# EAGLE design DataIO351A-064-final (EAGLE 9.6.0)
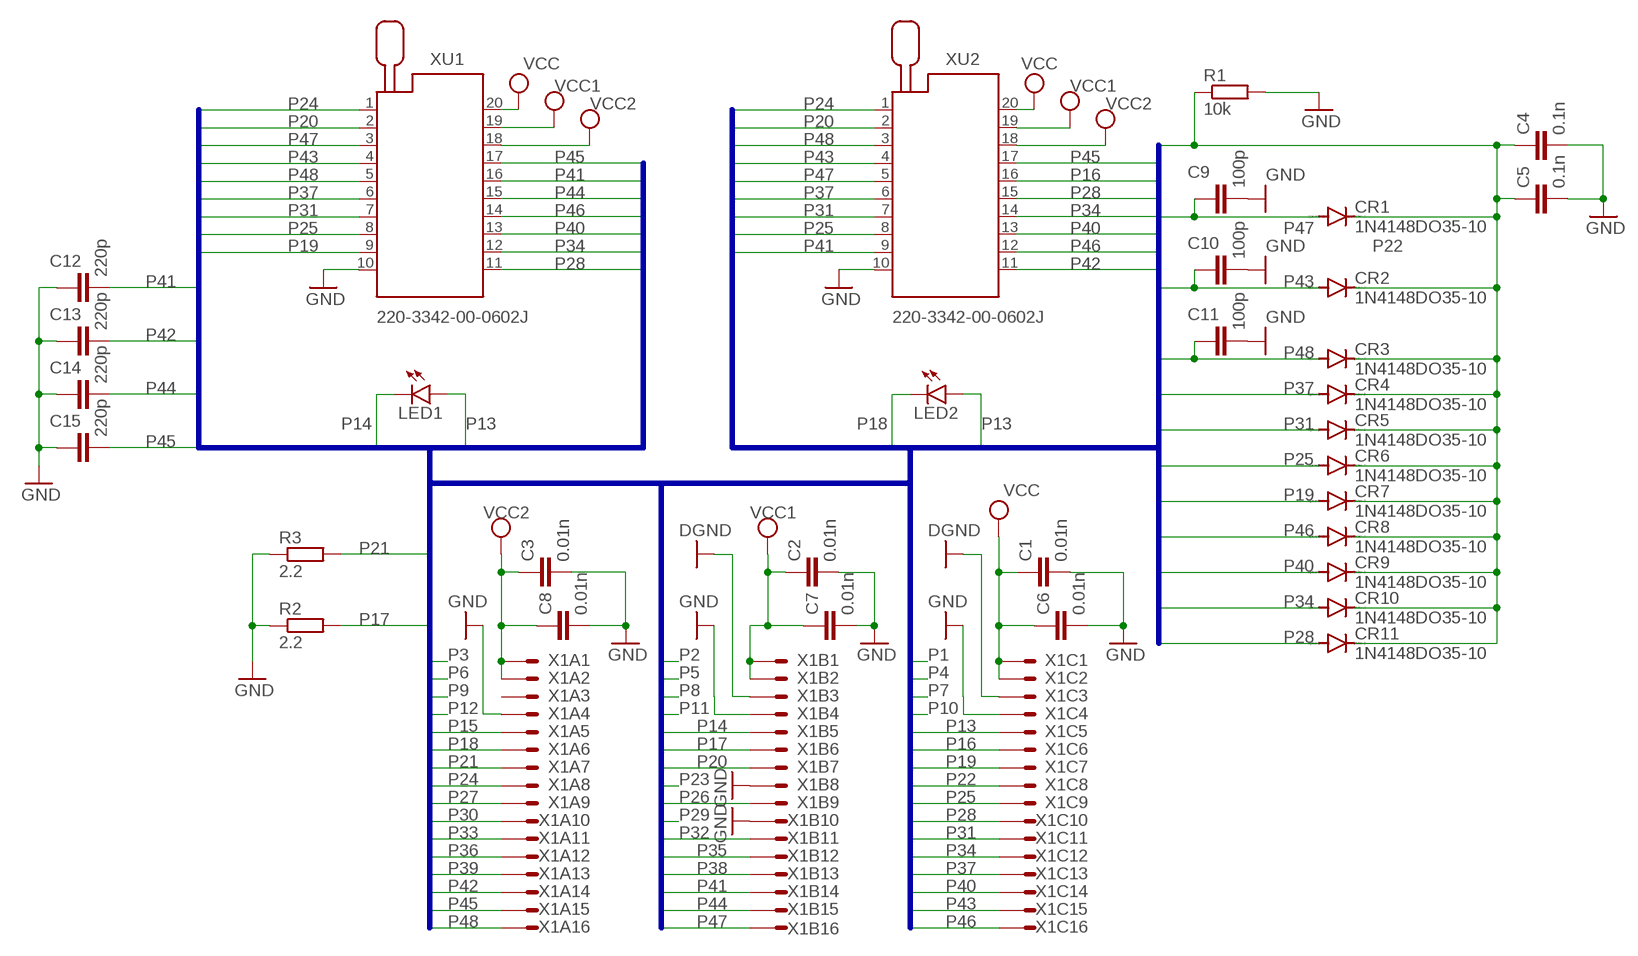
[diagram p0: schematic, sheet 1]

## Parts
C1  0.01n  C-EU050-025X075  [C050-025X075]
C2  0.01n  C-EU050-025X075  [C050-025X075]
C3  0.01n  C-EU050-025X075  [C050-025X075]
C4  0.1n  C-EU050-025X075  [C050-025X075]
C5  0.1n  C-EU050-025X075  [C050-025X075]
C6  0.01n  C-EU050-025X075  [C050-025X075]
C7  0.01n  C-EU050-025X075  [C050-025X075]
C8  0.01n  C-EU050-025X075  [C050-025X075]
C9  100p  C-EU050-025X075  [C050-025X075]
C10  100p  C-EU050-025X075  [C050-025X075]
C11  100p  C-EU050-025X075  [C050-025X075]
C12  220p  C-EU050-025X075  [C050-025X075]
C13  220p  C-EU050-025X075  [C050-025X075]
C14  220p  C-EU050-025X075  [C050-025X075]
C15  220p  C-EU050-025X075  [C050-025X075]
CR1  1N4148DO35-10  [DO35-10]
CR2  1N4148DO35-10  [DO35-10]
CR3  1N4148DO35-10  [DO35-10]
CR4  1N4148DO35-10  [DO35-10]
CR5  1N4148DO35-10  [DO35-10]
CR6  1N4148DO35-10  [DO35-10]
CR7  1N4148DO35-10  [DO35-10]
CR8  1N4148DO35-10  [DO35-10]
CR9  1N4148DO35-10  [DO35-10]
CR10  1N4148DO35-10  [DO35-10]
CR11  1N4148DO35-10  [DO35-10]
LED1  LED5MM  [LED5MM]
LED2  LED5MM  [LED5MM]
R1  10k  R-EU_V234/12  [V234/12]
R2  2.2  R-EU_V234/12  [V234/12]
R3  2.2  R-EU_V234/12  [V234/12]
X1  MAC48SHE  [MAC48SH]
XU1  220-3342-00-0602J  [220-3342-00-0602J]
XU2  220-3342-00-0602J  [220-3342-00-0602J]

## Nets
DGND: X1.B3 X1.C3
GND: C1.2 C2.2 C3.2 C4.2 C5.2 C6.2 C7.2 C8.2 C9.2 C10.2 C11.2 C12.1 C13.1 C14.1 C15.1 R1.2 R2.1 R3.1 X1.A4 X1.B4 X1.B8 X1.B10 X1.C4 XU1.10 XU2.10
P13: LED1.A LED2.A X1.C5
P14: LED1.K(C) X1.B5
P15: X1.A5
P16: X1.C6 XU2.16
P17: R2.2 X1.B6
P18: LED2.K(C) X1.A6
P19: CR7.A X1.C7 XU1.9
P20: X1.B7 XU1.2 XU2.2
P21: R3.2 X1.A7
P22: C4.1 C5.1 CR1.C CR2.C CR3.C CR4.C CR5.C CR6.C CR7.C CR8.C CR9.C CR10.C CR11.C R1.1 X1.C8
P24: X1.A8 XU1.1 XU2.1
P25: CR6.A X1.C9 XU1.8 XU2.8
P26: X1.B9
P27: X1.A9
P28: CR11.A X1.C10 XU1.11 XU2.15
P30: X1.A10
P31: CR5.A X1.C11 XU1.7 XU2.7
P32: X1.B11
P33: X1.A11
P34: CR10.A X1.C12 XU1.12 XU2.14
P35: X1.B12
P36: X1.A12
P37: CR4.A X1.C13 XU1.6 XU2.6
P38: X1.B13
P39: X1.A13
P40: CR9.A X1.C14 XU1.13 XU2.13
P41: C12.2 X1.B14 XU1.16 XU2.9
P42: C13.2 X1.A14 XU2.11
P43: C10.1 CR2.A X1.C15 XU1.4 XU2.4
P44: C14.2 X1.B15 XU1.15
P45: C15.2 X1.A15 XU1.17 XU2.17
P46: CR8.A X1.C16 XU1.14 XU2.12
P47: C9.1 CR1.A X1.B16 XU1.3 XU2.5
P48: C11.1 CR3.A X1.A16 XU1.5 XU2.3
VCC: C1.1 C6.1 X1.C1 X1.C2 XU1.20 XU2.20
VCC1: C2.1 C7.1 X1.B1 X1.B2 XU1.19 XU2.19
VCC2: C3.1 C8.1 X1.A1 X1.A2 XU1.18 XU2.18
Unconnected: X1.A3

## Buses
B:P[1..48]

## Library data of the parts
C1-C15 = rcl:C-EU: CAPACITOR, European symbol; SPICEPREFIX: C
CR1-CR11 = diode:1N4148: DIODE
LED1 LED2 = led:LED: LED
R1-R3 = rcl:R-EU_: RESISTOR, European symbol; SPICEPREFIX: R
X1 = con-vg:MAC48SHE: CONNECTOR male, 48 pins, single, type C/2, rows ABC, grid 2.54 mm
XU1 XU2 = con-3m:220-3342-00-0602J: Zero Insertion Force Socked Source: http://www.3M.com/ehpd; MF: 3M; MPN: 220-3342-00-0602J; OC_FARNELL: 9897445; OC_NEWARK: 85K7807

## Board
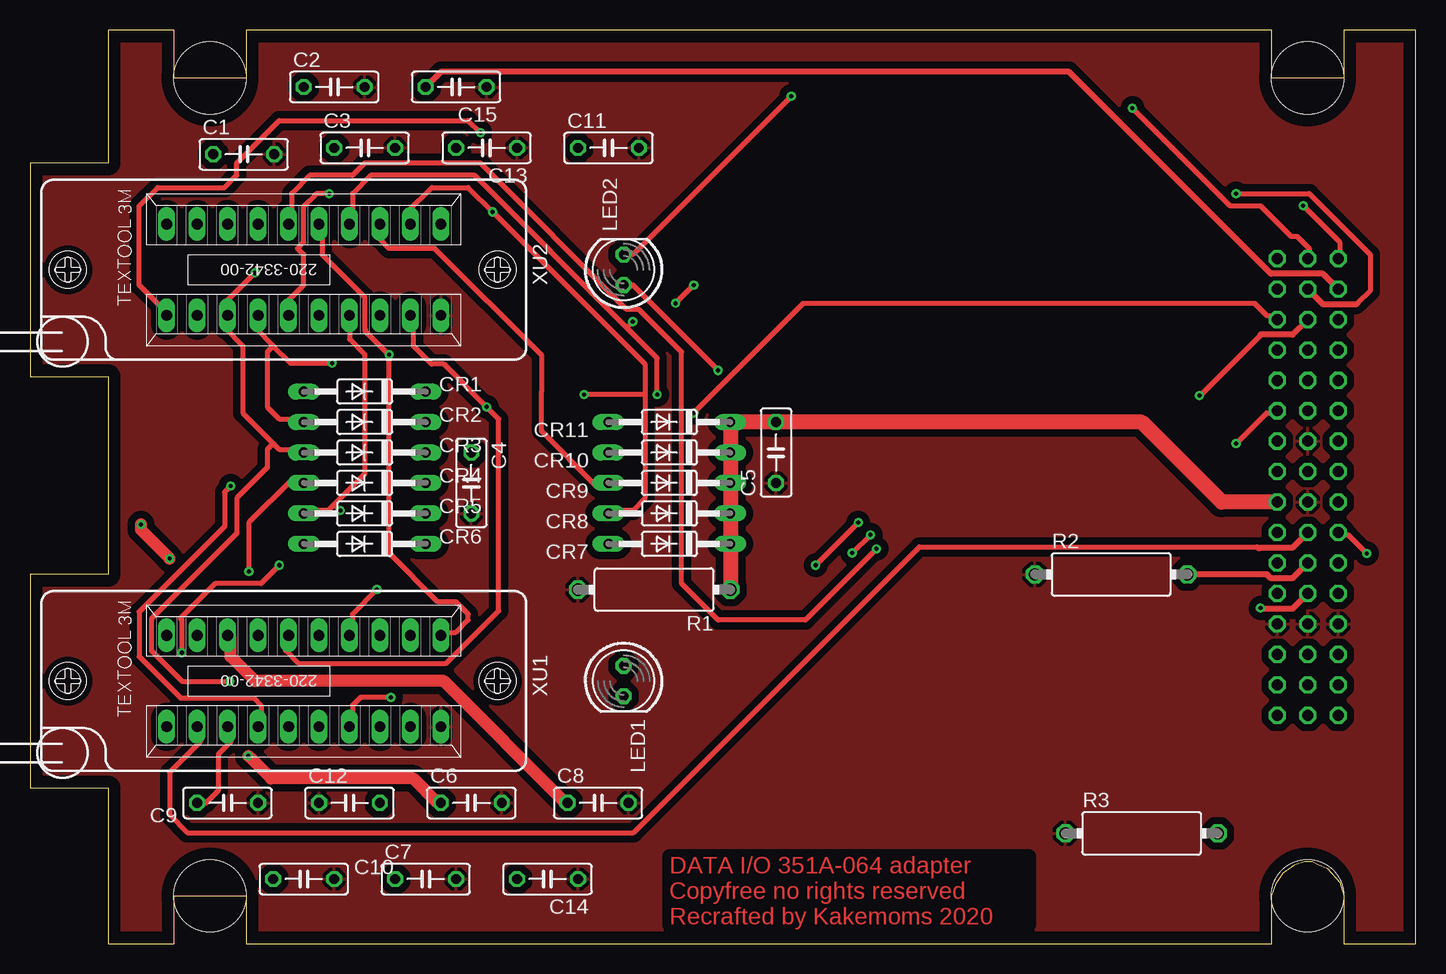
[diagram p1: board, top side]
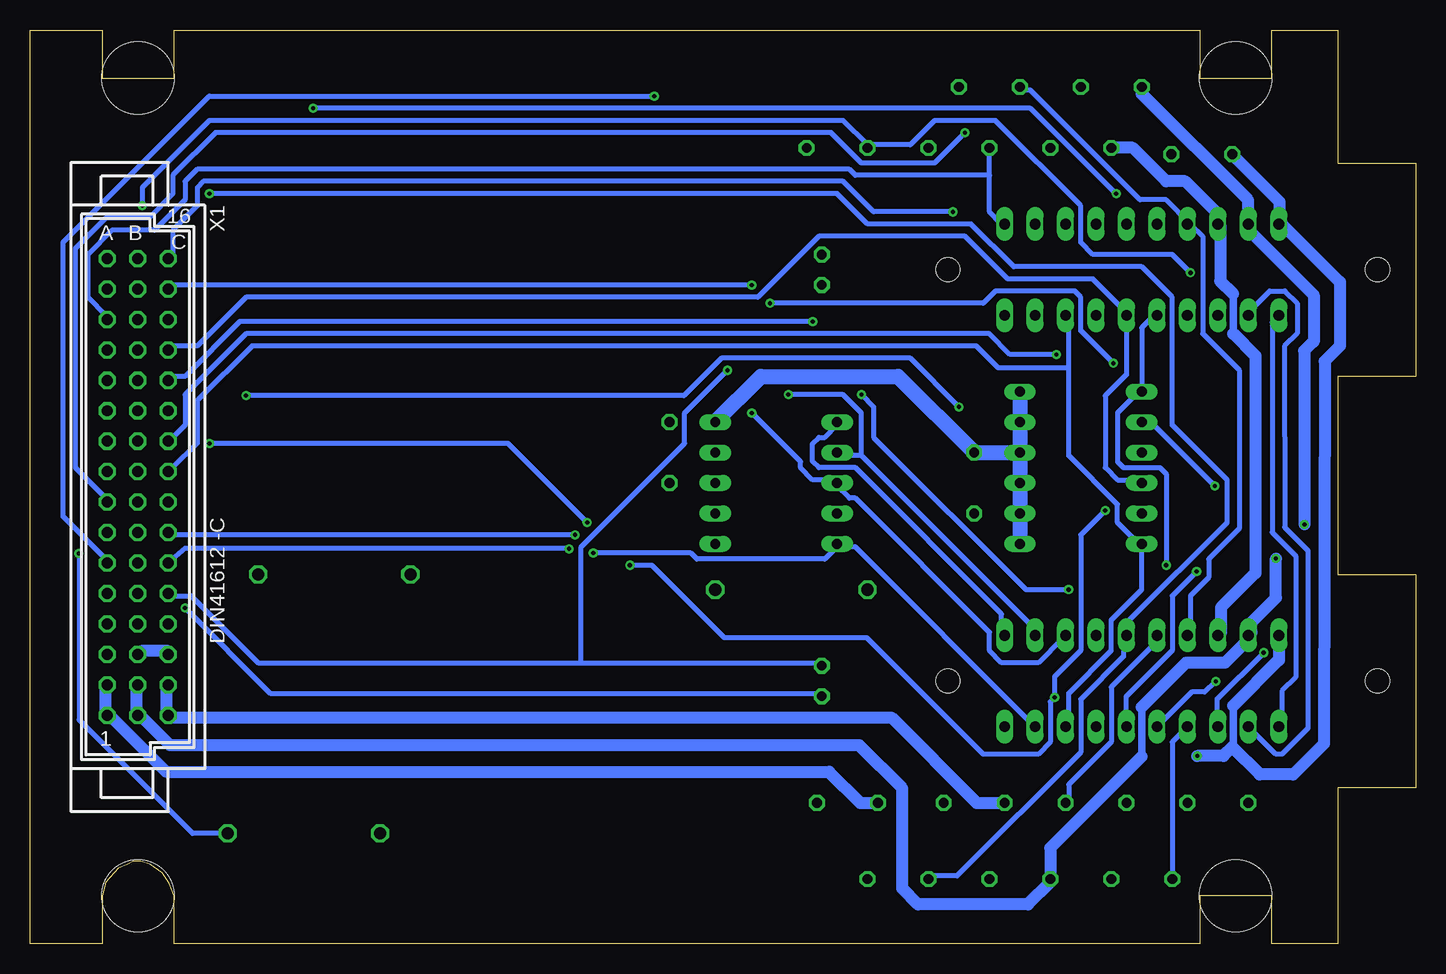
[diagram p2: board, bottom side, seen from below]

Size 115.5 x 76.2 mm. Coordinates in mm from the lower left corner, seen from the top.
Outline: 6.5,0 12,0 12,4 18,4 18,0 103.5,0 103.5,4 103.88,5.06 104.48,5.92 105.5,6.62 106.26,6.87 106.89,6.87 107.34,6.62 108.16,6.3 109.18,5.16 109.5,4 109.5,0 115.5,0 115.5,76.2 109.5,76.2 109.5,72.2 103.5,72.2 103.5,76.2 18,76.2 18,72.2 12,72.2 12,76.2 6.5,76.2 6.5,65.1 0,65.1 0,63.83 0,48.59 0,47.32 6.5,47.32 6.5,30.81 0,30.81 0,29.54 0,14.3 0,13.03 6.5,13.03 6.5,0
Copper layers (1*16): Top 0.035mm / dielectric 1.5mm / Bottom 0.035mm
Design rules "default *": minimum track width 16mil, minimum drill 0.35mm, track to track 24mil, track to pad 12mil, pad to pad 12mil, via to via 12mil, smd to smd 12mil, copper to edge 40mil, drill to drill 24mil, minimum pad ring 10mil, minimum via ring 8mil, stop-mask expansion 4mil, vias tented up to drill 0mil, thermal gap 12mil
Holes 6 mm at 106.5,4 106.5,72.2 15,4 15,72.2

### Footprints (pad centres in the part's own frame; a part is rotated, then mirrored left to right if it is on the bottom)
C050-025X075 = drill 0.813 octagon: 1 -2.54,0; 2 2.54,0
DO35-10 = drill 0.813 long: A 5.08,0; C -5.08,0
LED5MM = drill 0.813 octagon: A -1.27,0; K 1.27,0
V234/12 = drill 1.016 octagon: 1 -6.35,0; 2 6.35,0
MAC48SH = drill 0.914 octagon: A1 2.54,19.05; A2 2.54,16.51; A3 2.54,13.97; A4 2.54,11.43; A5 2.54,8.89; A6 2.54,6.35; A7 2.54,3.81; A8 2.54,1.27; A9 2.54,-1.27; A10 2.54,-3.81; A11 2.54,-6.35; A12 2.54,-8.89; A13 2.54,-11.43; A14 2.54,-13.97; A15 2.54,-16.51; A16 2.54,-19.05; B1 0,19.05; B2 0,16.51; B3 0,13.97; B4 0,11.43; B5 0,8.89; B6 0,6.35; B7 0,3.81; B8 0,1.27; B9 0,-1.27; B10 0,-3.81; B11 0,-6.35; B12 0,-8.89; B13 0,-11.43; B14 0,-13.97; B15 0,-16.51; B16 0,-19.05; C1 -2.54,19.05; C2 -2.54,16.51; C3 -2.54,13.97; C4 -2.54,11.43; C5 -2.54,8.89; C6 -2.54,6.35; C7 -2.54,3.81; C8 -2.54,1.27; C9 -2.54,-1.27; C10 -2.54,-3.81; C11 -2.54,-6.35; C12 -2.54,-8.89; C13 -2.54,-11.43; C14 -2.54,-13.97; C15 -2.54,-16.51; C16 -2.54,-19.05
220-3342-00-0602J = drill 0.9 long: 1 -11.43,-3.81; 2 -8.89,-3.81; 3 -6.35,-3.81; 4 -3.81,-3.81; 5 -1.27,-3.81; 6 1.27,-3.81; 7 3.81,-3.81; 8 6.35,-3.81; 9 8.89,-3.81; 10 11.43,-3.81; 11 11.43,3.81; 12 8.89,3.81; 13 6.35,3.81; 14 3.81,3.81; 15 1.27,3.81; 16 -1.27,3.81; 17 -3.81,3.81; 18 -6.35,3.81; 19 -8.89,3.81; 20 -11.43,3.81 | hole 2: 16.16,0; -19.66,0

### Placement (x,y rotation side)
C1  17.82,65.84 0 top
C2  25.36,71.45 0 top
C3  27.9,66.37 0 top
C4  36.79,38.43 270 top
C5  62.19,40.97 270 top
C6  36.79,11.76 0 top
C7  32.98,5.41 0 top
C8  47.36,11.76 0 top
C9  16.47,11.76 0 top
C10  22.82,5.41 0 top
C11  48.22,66.37 0 top
C12  26.63,11.76 0 top
C13  38.06,66.37 180 top
C14  43.14,5.41 180 top
C15  35.52,71.45 180 top
CR1  27.9,46.05 180 top
CR2  27.9,43.51 180 top
CR3  27.9,40.97 180 top
CR4  27.9,38.43 180 top
CR5  27.9,35.89 180 top
CR6  27.9,33.35 180 top
CR7  53.3,33.35 180 top
CR8  53.3,35.89 180 top
CR9  53.3,38.43 180 top
CR10  53.3,40.97 180 top
CR11  53.3,43.51 180 top
LED1  49.49,21.92 270 top
LED2  49.49,56.21 90 top
R1  52.03,29.54 180 top
R2  90.13,30.81 0 top
R3  92.67,9.22 0 top
X1  106.51,38.1 180 bottom
XU1  22.82,21.92 0 top
XU2  22.82,56.21 0 top

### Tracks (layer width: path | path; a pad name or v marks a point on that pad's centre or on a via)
DGND
  Bottom 0.406: 104.1,24.46 X1.C3 | 106.13,24.46 X1.B3
  Bottom 1.016: 106.13,24.46 104.1,24.46
GND
  pour Top: 0.21,76.53 115.53,76.53 115.53,-0.03 0.21,-0.03
P13  (via drill 0.35)
  Top 0.406: v57.36,47.83 50.25,54.94 49.74,54.94 LED2.A
  Bottom 0.406: 69.56,23.44 96.48,23.44 102.07,29.03 103.59,29.03 X1.C5 | 69.56,23.44 49.74,23.44 LED1.A | v57.36,47.83 60.92,44.27 60.92,41.73 69.56,33.1 69.56,23.44
P14  (via drill 0.35)
  Top 0.406: v102.58,28.02 102.58,27.94
  Top 0.508: X1.B5 105.24,27.94 102.58,27.94 102.42,27.94
  Bottom 0.406: v102.58,28.02 95.46,20.9 49.74,20.9 LED1.K
P16  (via drill 0.35)
  Top 0.406: v70.57,32.94 64.63,27 57.36,27 54.32,30.05 54.32,49.35 50.76,52.91 49.74,52.91 37.55,65.1 27.9,65.1 26.88,64.08 23.33,64.08 21.8,62.56 21.8,60.02 XU2.16
  Bottom 0.406: v70.57,32.94 70.62,32.99 102.54,32.99 X1.C6
P17
  Top 0.508: R2.2 103.12,30.81 103.45,30.48 105.24,30.48 X1.B6
P18  (via drill 0.35)
  Top 0.406: v63.46,70.69 50.25,57.48 49.74,57.48 LED2.K
  Bottom 0.406: v63.46,70.69 100.54,70.69 112.74,58.5 112.74,35.64 109.18,32.08 X1.A6
P19  (via drill 0.35)
  Top 0.406: v68.54,32.59 v70.06,34.11
  Bottom 0.406: 48.22,33.1 46.7,33.1 31.96,18.36 XU1.9 | 48.22,33.1 CR7.A 48.22,33.1 | v70.06,34.11 103.59,34.11 X1.C7 | v68.54,32.59 60.41,32.59 59.9,32.08 49.24,32.08 48.22,33.1
P20
  Top 0.406: 102.37,33.02 102.3,33.1 74.13,33.1 50.3,9.27 13.12,9.27 11.64,10.74 11.64,14.3 14.18,16.84 14.18,17.86 XU1.2
  Top 0.508: X1.B7 105.24,33.02 102.58,33.02 102.37,33.02
  Bottom 0.406: XU1.2 13.68,17.86 11.64,15.82 11.14,15.82 8.98,17.98 8.98,32.79 10.91,34.72 10.93,49.84 9.87,50.9 9.87,53.42 10.88,54.43 10.91,54.43 12.15,54.43 13.85,52.73 13.93,52.73 XU2.2
P21  (via drill 0.35)
  Top 0.406: v111.44,32.56 109.89,34.11 109.18,34.11 X1.A7
  Bottom 0.406: v111.44,32.56 111.42,32.54 111.42,18.69 101.94,9.22 R3.2
P22
  Top 0.406: 58.38,33.6 CR7.C | 58.38,36.14 CR8.C | 58.38,38.68 CR9.C | 58.38,41.22 CR10.C
  Top 1.27: X1.C8 99.35,36.83 92.67,43.51 C5.1 CR11.C 58.38,41.22 CR10.C 58.38,38.68 CR9.C 58.38,36.14 CR8.C 58.38,33.6 CR7.C R1.1
  Bottom 0.406: 32.98,36.14 CR5.C | 32.98,38.18 CR4.C | 32.98,43.76 CR2.C
  Bottom 1.27: CR11.C 54.57,47.32 43.14,47.32 C4.1 CR3.C | CR1.C 32.98,43.76 CR2.C CR3.C | CR3.C CR4.C 32.98,38.18 32.98,36.14 CR5.C CR6.C
P24  (via drill 0.35)
  Top 0.406: v37.55,67.64 36.54,68.66 20.79,68.66 17.23,65.1 17.23,64.08 16.22,63.07 10.63,63.07 9.1,61.54 9.1,54.94 11.64,52.4 XU2.1
  Bottom 0.406: XU2.1 11.95,51.84 11.95,34.32 9.99,32.36 9.99,22.23 11.14,21.08 11.14,18.36 XU1.1 | v37.55,67.64 40.09,65.1 46.19,65.1 48.73,67.64 100.04,67.64 103.59,64.08 103.59,62.56 105.62,60.53 109.18,60.53 111.72,57.99 111.72,39.7 109.18,37.16 X1.A8
P25
  Bottom 0.406: 22.82,33.1 22.82,29.54 25.36,27 25.36,24.46 28.92,20.9 28.92,18.36 XU1.8 | 22.82,33.1 CR6.A 22.82,33.1 | 28.92,48.03 28.92,40.72 24.85,36.65 24.85,35.13 22.82,33.1 | 28.92,48.03 28.92,48.84 28.92,52.4 XU2.8 | 28.92,48.03 34.78,48.03 36.61,49.86 96.99,49.86 101.56,45.29 101.56,41.73 103.59,39.7 X1.C9
P28  (via drill 0.35)
  Top 0.406: XU2.15 24.34,60.02 24.34,57.48 27.9,53.92 27.9,51.3 | XU1.11 34.5,25.98 35.52,25.98 36.54,27 36.54,27.51 35.52,28.52 34,28.52 29.93,32.59 29.93,46.81 v29.93,49.15 29.88,49.15 27.9,51.13 27.9,51.3 | 27.96,51.24 27.9,51.3
  Bottom 0.406: CR11.A 48.22,43.26 49.24,42.24 49.74,42.24 50.25,41.73 50.25,40.21 49.74,39.7 46.7,39.7 34.5,27.51 34.5,25.98 XU1.11 | v29.93,49.15 33.79,49.15 35.52,50.88 97.5,50.88 102.58,45.8 102.58,43.26 103.59,42.24 X1.C10
P31  (via drill 0.35)
  Top 0.406: 25.36,36.65 27.9,39.19 27.9,49.15 26.63,50.42 XU2.7 | 25.36,36.65 24.85,36.14 22.82,36.14 CR5.A | v30.08,20.55 30.06,20.57 27.57,20.57 26.88,19.89 26.88,18.36 XU1.7 | 25.36,36.65 v25.87,36.14 | v100.54,41.73 103.08,44.27 103.59,44.27 X1.C11 | v65.49,31.57 v69.05,35.13
  Bottom 0.406: v25.87,36.14 27.9,34.11 27.9,24.46 30.08,22.28 v30.08,20.55 30.44,20.19 30.44,16.84 31.46,15.82 36.03,15.82 45.73,25.53 57.62,25.53 63.66,31.57 v65.49,31.57 | v100.54,41.73 75.65,41.73 v69.05,35.13
P34  (via drill 0.35)
  Top 0.406: 49.74,51.38 52.28,48.84 v52.28,45.8 | 49.74,51.38 37.04,64.08 28.41,64.08 26.88,62.56 26.88,60.02 XU2.14 | 49.74,51.38 v50.25,51.89
  Bottom 0.406: 46.19,40.72 48.22,40.72 CR10.A | 46.19,40.72 31.46,25.98 XU1.12 | v52.28,45.8 47.71,45.8 46.19,44.27 46.19,40.72 | v50.25,51.89 98,51.89 102.58,47.32 103.59,47.32 X1.C12
P37  (via drill 0.35)
  Top 0.406: v18.25,31.06 18.25,35.13 21.8,38.68 22.82,38.68 CR4.A
  Bottom 0.406: CR4.A 22.82,38.68 24.85,38.68 25.87,39.7 25.87,45.72 24.17,47.42 24.11,47.42 24.09,47.45 XU2.6 23.84,52.4 26.88,55.45 34,55.45 37.55,59 49.74,59 54.82,53.92 97.5,53.92 101.56,49.86 103.59,49.86 X1.C13 | XU1.6 24.14,18.16 24.14,20.6 20.28,24.46 20.28,29.03 v18.25,31.06
P40  (via drill 0.35)
  Top 0.406: XU2.13 29.17,58.75 29.93,57.99 33.74,57.99 42.63,49.1 42.63,46.05 42.63,42.75 47.2,38.18 48.22,38.18 CR9.A | v55.33,44.27 64.48,53.42 102.07,53.42 103.08,52.4 103.59,52.4 X1.C14
  Bottom 0.406: XU1.13 29.42,25.48 31.46,23.44 34.5,23.44 35.52,24.46 35.52,25.98 46.7,37.16 47.2,37.16 48.22,38.18 CR9.A 48.22,38.68 50.25,38.68 51.27,39.7 51.27,40.21 v55.33,44.27
P41  (via drill 0.35)
  Top 0.406: XU2.9 31.96,52.4 31.96,49.86 33.49,48.34 34.5,48.34 v38.06,44.78 39.08,43.76 39.08,27.76 34.71,23.39 22.36,23.39 21.3,24.46 21.3,25.48 XU1.16 | 102.58,50.8 102.58,50.72 97.57,45.72 v97.5,45.72 | 102.58,50.8 102.58,50.88 102.58,50.8
  Top 0.508: X1.B14 105.24,50.8 102.58,50.8
  Bottom 0.406: C12.2 28.92,11.76 28.92,13.28 25.36,16.84 25.36,21.41 21.3,25.48 XU1.16 | v97.5,45.72 61,45.72 57.87,48.84 42.12,48.84 v38.06,44.78
P42
  Bottom 0.406: 35.52,64.08 35.52,61.04 34.5,60.02 XU2.11 | 35.52,64.08 35.52,66.12 C13.2 | 35.52,64.08 46.7,64.08 47.2,64.59 101.56,64.59 102.58,63.58 102.58,62.05 105.12,59.51 108.67,59.51 110.7,57.48 110.7,53.92 109.18,52.4 X1.A14
P43  (via drill 0.35)
  Top 0.406: 20.28,49.86 19.77,49.35 19.77,44.78 20.79,43.76 22.82,43.76 CR2.A | 20.28,49.86 18.76,51.38 18.76,52.4 XU2.4 | v53.81,53.42 v55.33,54.94 | v25.18,48.41 21.73,48.41 20.28,49.86 | v16.72,38.18 16.22,37.67 16.22,34.8 9.1,27.69 9.1,23.95 12.56,20.5 18.63,20.5 19.26,19.86 19.26,18.36 XU1.4
  Bottom 0.406: C10.1 20.28,5.66 20.28,16.84 19.26,17.86 XU1.4 | v55.33,54.94 103.59,54.94 X1.C15 | v53.81,53.42 36.03,53.42 35.01,54.43 28.41,54.43 27.9,53.92 27.9,51.13 v25.18,48.41 | v16.72,38.18 21.8,43.26 22.82,43.26 CR2.A
P44  (via drill 0.35)
  Top 0.406: v100.54,62.56 106.64,62.56 111.72,57.48 111.72,54.43 110.7,53.42 110.53,53.34
  Top 0.508: X1.B15 107.78,53.34 110.53,53.34
  Bottom 0.406: C14.2 40.6,5.66 38.21,5.66 27.9,15.98 27.9,20.4 24.34,23.95 24.34,25.48 XU1.15 23.84,25.98 23.84,27 15.71,35.13 15.71,38.68 20.28,43.26 20.28,53.92 22.82,56.46 33.49,56.46 37.04,60.02 45.68,60.02 48.22,62.56 v100.54,62.56
P45
  Top 0.508: X1.A15 107.78,55.88 103.45,55.88 86.61,72.72 34.25,72.72 C15.2
  Bottom 0.406: 18.76,60.02 20.79,62.05 22.97,62.05 32.12,71.2 32.98,71.2 C15.2 | 18.76,60.02 XU2.17 18.76,60.02 | 18.76,60.02 17.74,59 17.74,50.88 14.69,47.83 14.69,34.62 17.23,32.08 17.23,30.56 18.76,29.03 18.76,25.98 XU1.17
P46  (via drill 0.35)
  Top 0.406: 51.27,45.8 51.27,48.34 v38.57,61.04 36.54,63.07 33.49,63.07 31.46,61.04 31.46,60.02 XU2.12 | 51.27,45.8 51.27,37.16 50.25,36.14 48.22,36.14 CR8.A | v28.92,29.54 26.88,27.51 26.88,25.98 XU1.14 | 51.27,45.8 v46.19,45.8
  Bottom 0.406: v28.92,29.54 32.47,29.54 45.17,42.24 45.17,44.78 v46.19,45.8 | v38.57,61.04 45.17,61.04 47.71,63.58 101.05,63.58 101.56,63.07 101.56,61.54 103.59,59.51 103.59,57.48 X1.C16
P47  (via drill 0.35)
  Top 0.406: C9.1 14.18,11.76 14.69,11.76 15.71,12.78 15.71,15.82 16.72,16.84 16.72,17.86 XU1.3 | v91.91,69.67 100.04,61.54 102.58,61.54 105.12,59 105.62,59 106.64,57.99 106.64,57.48 X1.B16 | v24.95,62.56 24.93,62.54 23.86,62.54 23.81,62.48 22.82,61.49 22.82,58.5 22.31,57.99 22.82,57.48 22.82,54.94 21.3,53.42 21.3,52.4 XU2.5 | v12.66,24.28 12.66,27 12.53,27.13 15.45,30.05 19.26,30.05 v20.79,31.57
  Bottom 0.406: 22.82,46.3 22.82,51.38 21.8,52.4 XU2.5 | 22.82,46.3 CR1.A 22.82,46.3 | v91.91,69.67 32.09,69.67 24.98,62.56 v24.95,62.56 | XU1.3 16.55,18.19 16.55,20.4 v12.66,24.28 | v20.79,31.57 20.79,39.19 21.3,39.7 24.34,39.7 24.85,40.21 24.85,44.27 22.82,46.3
P48  (via drill 0.35)
  Top 0.406: 20.28,41.73 17.74,44.27 17.74,49.86 16.22,51.38 16.22,52.4 | 20.28,41.73 20.79,41.22 22.82,41.22 CR3.A | 16.22,52.4 XU2.3 16.22,52.4 | v18.76,55.96 16.22,53.42 16.22,52.4 | v16.65,21.9 12.69,21.9 10.12,24.46 10.12,27.1 17.23,34.21 17.23,37.16 19.77,39.7 19.77,41.22 20.28,41.73 | v106.13,61.54 109.18,58.5 109.18,57.48 X1.A16
  Bottom 0.406: 45.68,66.62 42.12,66.62 40.09,68.66 35.01,68.66 27.9,61.54 27.9,58.5 26.88,57.48 20.28,57.48 v18.76,55.96 | 45.68,66.62 C11.1 45.68,66.62 | v16.65,21.9 16.7,21.9 17.59,21.01 18.65,21.01 21.3,18.36 XU1.5 | v106.13,61.54 106.13,63.07 100.54,68.66 47.71,68.66 45.68,66.62
VCC  (via drill 0.35)
  Top 0.406: 34,11.76 C6.1
  Top 1.016: 34,11.76 31.96,13.79 20.1,13.79 18.22,15.67 v18.2,15.67
  Bottom 0.406: 11.14,60.02 XU2.20 | 34.5,11.76 C6.1 | 103.59,18.87 X1.C1 104.1,19.38 | 104.1,21.41 X1.C2
  Bottom 0.61: 15.2,16.33 15.2,19.86
  Bottom 1.016: C1.1 15.28,65.81 11.31,61.85 11.31,60.1 XU2.20 | XU1.20 11.39,23.67 15.2,19.86 | 15.28,16.41 12.99,14.12 10.2,14.12 7.63,16.69 7.58,48.59 6.31,49.86 6.31,55.19 11.14,60.02 | 15.28,16.41 15.2,16.33 | 34.5,11.76 36.59,11.76 43.7,18.87 103.59,18.87 | 104.1,19.38 104.1,21.41 | v18.2,15.67 16.01,15.67 15.28,16.41
VCC1  (via drill 0.35)
  Top 1.016: v11.64,32.13 9.26,34.52 v9.26,34.98
  Bottom 0.406: 22.82,71.2 C2.1 | 13.96,60.02 XU2.19 13.68,60.02 13.68,59.28 | 106.64,19.38 X1.B1 106.13,18.87 | 106.64,21.41 X1.B2 | 30.44,5.66 C7.1 30.44,5.16 | 14.18,25.48 XU1.19 13.68,25.98
  Bottom 0.61: 22.82,19.76 22.82,15.62
  Bottom 1.016: 22.82,71.2 22.82,70.87 13.96,62 13.96,60.02 | 106.64,21.41 106.64,19.38 | 30.44,5.66 30.44,8 22.82,15.62 | 22.82,19.76 19.14,23.44 15.89,23.44 14.18,25.15 14.18,25.48 | 106.13,18.87 103.82,16.56 46.39,16.56 42.78,12.95 42.78,4.62 41.46,3.3 32.29,3.3 30.44,5.16 | 13.68,59.28 8.49,54.1 8.49,50.19 8.54,50.19 9.28,49.45 v9.26,34.98 | v11.64,32.13 11.64,28.85 13.68,26.82 13.68,25.98
VCC2
  Top 0.406: 16.72,25.48 XU1.18 | 44.66,11.76 C8.1
  Top 1.016: 16.72,25.48 16.72,23.95 18.76,21.92 34.5,21.92 44.66,11.76
  Bottom 0.406: 16.32,60.71 16.32,60.12 16.22,60.02 XU2.18 | 16.22,25.98 XU1.18 | 109.18,21.92 X1.A2 109.18,21.41 | 44.66,11.76 C8.1 | 108.67,18.87 X1.A1 109.18,19.38
  Bottom 0.61: 16.27,55.35 16.29,55.3 | 15.2,54.2 15.2,50.88
  Bottom 1.016: C3.1 23.58,66.37 20.79,63.58 19.19,63.58 16.32,60.71 | 16.22,25.98 16.22,28.04 13.35,30.91 13.35,49.02 15.2,50.88 | 16.29,55.3 15.2,54.2 | XU2.18 16.27,59.82 16.27,55.35 | 44.66,11.76 46.29,11.76 48.88,14.35 104.15,14.35 108.67,18.87 | 109.18,19.38 109.18,21.41

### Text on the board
Top: DATA I/O 351A-064 adapter / Copyfree no rights reserved / Recrafted by Kakemoms 2020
